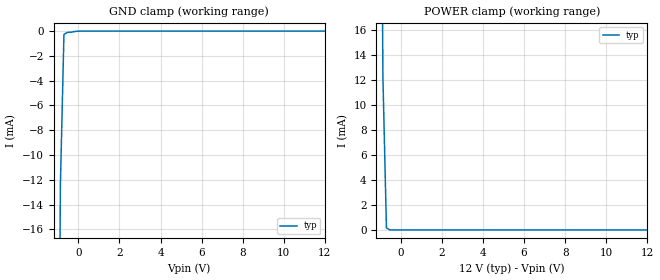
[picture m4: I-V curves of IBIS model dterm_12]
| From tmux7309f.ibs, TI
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| dterm_12
[Model]   dterm_12
Model_type   Terminator
|   typ   min   max
C_comp   1.008417e-11   NA   NA
[Voltage Range]   12   NA   NA
[Temperature Range]   27   NA   NA
[Power Clamp Reference]   12   NA   NA
[GND Clamp Reference]   0   NA   NA
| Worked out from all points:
|   GND clamp passes 1 mA (typ) near -0.72 V on its own axis
|   POWER clamp passes 1 mA (typ) near -0.72 V on its own axis
[GND Clamp]
|   Voltage   I(typ)   I(min)   I(max)
-5V       -1.414A    NA         NA
-1.051V   -55.81mA   NA         NA
-878.8mV  -12.35mA   NA         NA
-707.1mV  -268.4uA   NA         NA
-535.4mV  -103.8uA   NA         NA
151.5mV   -38.17nA   NA         NA
12V       2.395nA    NA         NA
[POWER Clamp]
|   Voltage   I(typ)   I(min)   I(max)
-5V       1.414A     NA         NA
-1.05V    55.75mA    NA         NA
-878.8mV  12.22mA    NA         NA
-707.1mV  161.7uA    NA         NA
-535.4mV  644nA      NA         NA
12V       -4.134uA   NA         NA
